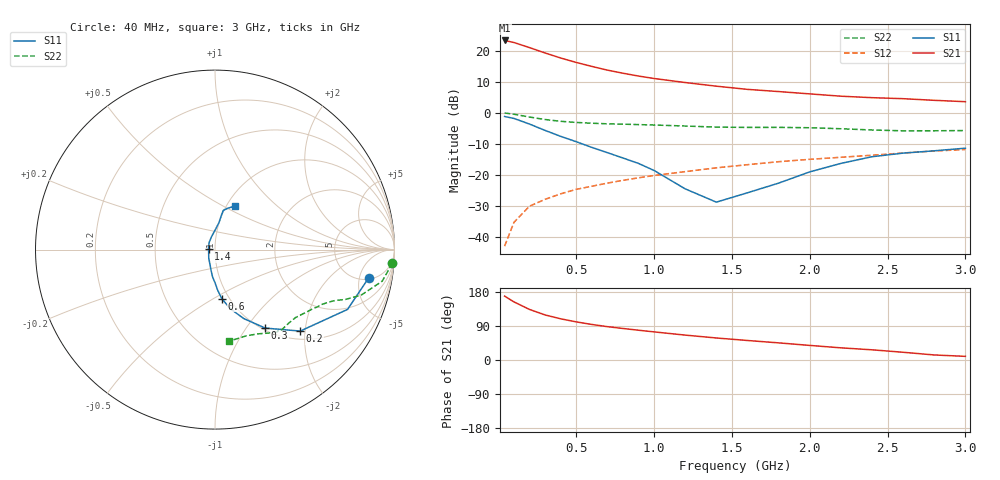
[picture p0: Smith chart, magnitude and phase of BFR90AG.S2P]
! Filename:  BFR90AG.S2P  Version:  2.0
! Philips part #: BFR90A  Date: Jul 1990
! Bias condition: Vce=10V,  Ic=5mA
#  MHz  S  MA  R  50
! Freq  S11  S21  S12  S22  !GUM [dB]
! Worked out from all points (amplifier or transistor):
!   21 points, 40 MHz to 3 GHz, reference 50 ohm
!   highest |S21| = 23.4 dB at 40 MHz (marker M1)
!   |S21| within 3 dB of that: start of sweep to 239.7 MHz
!   unconditionally stable (mu >= 1): 892.5 MHz to end of sweep
!   at 300 MHz: K = 0.63, MSG = 23.6 dB, |S12| = -28.0 dB
!   at 1 GHz: K = 1.03, MAG = 14.7 dB, |S12| = -20.3 dB
!   at 3 GHz: K = 1.01, MAG = 7.0 dB, |S12| = -11.9 dB
!   S11 on the Smith chart (normalised r, x): 40 MHz: 5.33, -6.95; 200 MHz: 1.18, -1.88; 300 MHz: 1.03, -1.23; 600 MHz: 0.92, -0.55; 1.4 GHz: 0.93, +0.01; 3 GHz: 1.10, +0.57
40  0.871 -10.4  14.73 168.6  0.007 86.3  0.991 -4.4
100  0.81 -24.3  13.65 153.3  0.017 76.0  0.948 -10.7
200  0.657 -43.7  11.29 133.4  0.031 68.5  0.853 -17.3
300  0.519 -57.4  9.246 118.9  0.04 64.5  0.778 -20.9
400  0.416 -67.4  7.669 108.7  0.049 63.1  0.728 -22.9
500  0.341 -75.4  6.504 100.6  0.058 62.6  0.698 -24.8
600  0.276 -82.1  5.611 93.8  0.065 62.3  0.678 -26.4
700  0.227 -86.2  4.887 88.0  0.073 61.9  0.663 -27.7
800  0.186 -89.8  4.355 83.2  0.081 61.6  0.655 -29.1
900  0.152 -95.2  3.92 78.6  0.089 60.9  0.644 -30.3
1000  0.117 -100.9  3.58 74.2  0.097 60.2  0.634 -31.6
1200  0.059 -126.0  3.079 65.7  0.112 58.0  0.611 -35.4
1400  0.036 173.0  2.69 58.1  0.129 55.7  0.587 -40.2
1600  0.051 130.3  2.388 51.5  0.145 54.3  0.58 -45.2
1800  0.073 106.1  2.202 45.2  0.162 52.2  0.581 -49.9
2000  0.111 89.1  2.019 38.5  0.177 49.3  0.573 -53.4
2200  0.152 81.6  1.853 32.1  0.191 47.1  0.552 -57.4
2400  0.195 79.4  1.754 26.9  0.206 44.4  0.527 -63.0
2600  0.223 78.1  1.689 20.4  0.224 41.4  0.511 -70.1
2800  0.243 72.2  1.589 13.3  0.241 38.6  0.512 -76.5
3000  0.268 65.0  1.51 9.6  0.255 36.8  0.516 -81.3
